TYPE ST_SlaveStateInfo :
STRUCT
	nIndex 			: DINT;
	sName 			: STRING; 		(* name of slave given in System Manager *)
	sType 			: STRING;		(* type of slave, e.g. EK1100*)
	nECAddr 		: UINT;			(* EtherCAT Slave Addr *)
	bDiagData		: BOOL;			(* DiagData in Slave State *)
	stPortCRCErrors	: ST_EcCrcErrorEx;(* Slave CRC-Errors, separate for each Port *)
	nSumCRCErrors	: UDINT;		(* Slave CRC-Errors, sum of all Ports *)
	stState 		: ST_SlaveState;(* EtherCAT State and Link state*)
END_STRUCT
END_TYPE
